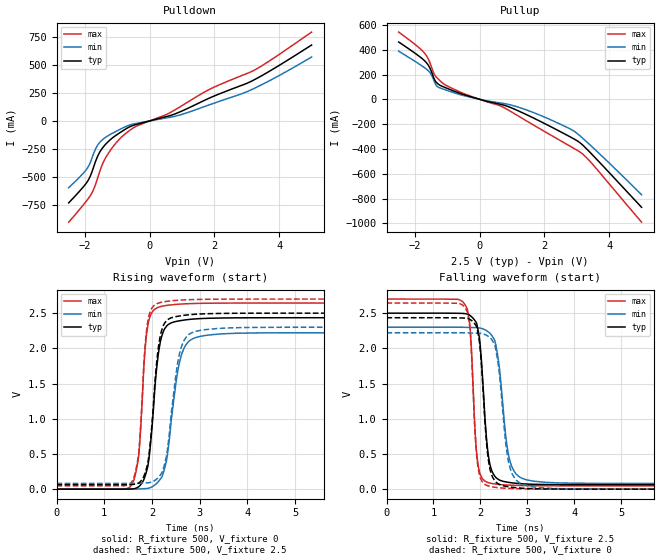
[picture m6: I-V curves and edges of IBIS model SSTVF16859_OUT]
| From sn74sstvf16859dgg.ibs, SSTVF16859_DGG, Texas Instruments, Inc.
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[Model]   SSTVF16859_OUT
Model_type  Output
Vref =   0
Rref =   500
Cref =   30p
Vmeas =   1.25
| variable   typ   min   max
C_comp   3.96pF   0.40pF   6.75pF
| C_pullup   3.64pF   0.40pF   6.75pF
| C_pulldown   4.29pF   2.35pF   5.77pF
[Temperature Range]   40   85   0
| Ambient temperature   25   70   0
[Voltage range]   2.5   2.3   2.7
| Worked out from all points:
|   slope of the pulldown table from 0 to 0.375 V, typ, clamps not added: 13.2 ohm
|   slope of the pullup table from 0 to 0.375 V, typ, clamps not added: 14.9 ohm
|   rising waveform, R_fixture 500, V_fixture 0: 20-80 % time 194ps typ, 256ps min, 144ps max; typ from 0 V to 2.44 V
|   falling waveform, R_fixture 500, V_fixture 2.5: 20-80 % time 156ps typ, 211ps min, 119ps max; typ from 2.5 V to 0.063 V
|   rising waveform, R_fixture 500, V_fixture 2.5: 20-80 % time 187ps typ, 239ps min, 142ps max; typ from 0.063 V to 2.5 V
|   falling waveform, R_fixture 500, V_fixture 0: 20-80 % time 155ps typ, 205ps min, 119ps max; typ from 2.44 V to 0 V
[Pulldown]
| SSTVF16859_OUT
|   Voltage   I(typ)   I(min)   I(max)
-2.5V     -732mA     -596.8mA   -904.7mA
-1.905V   -533.6mA   -413.3mA   -697.5mA
-1.725V   -407.4mA   -288.3mA   -608.5mA
-1.525V   -271.1mA   -186.6mA   -438mA
-1.215V   -167.6mA   -120.4mA   -263.3mA
-720mV    -68.68mA   -47.92mA   -107.3mA
-405mV    -31.09mA   -21.89mA   -46.25mA
935mV     80.65mA    53.1mA     125.3mA
1.84V     203.5mA    143.7mA    281mA
2.855V    319.5mA    243.8mA    406.9mA
3.48V     407.3mA    326.4mA    495.7mA
5V        678.2mA    571.1mA    793.7mA
[Pullup]
| SSTVF16859_OUT
|   Voltage   I(typ)   I(min)   I(max)
-2.5V     462.1mA    388.2mA    541.8mA
-1.72V    315.6mA    258.5mA    377.6mA
-1.52V    242.9mA    210.1mA    284.3mA
-1.355V   142.5mA    119.4mA    184.8mA
-1.095V   98.22mA    79.55mA    121.5mA
-455mV    34.94mA    27.86mA    42.59mA
715mV     -44.8mA    -32.33mA   -61.98mA
1.625V    -145.9mA   -103.1mA   -201.5mA
2.865V    -312.4mA   -248.6mA   -388.9mA
3.15V     -361.4mA   -306.3mA   -434.6mA
3.41V     -428.1mA   -367.8mA   -500.6mA
5V        -870.5mA   -768.8mA   -990.2mA
[Ramp]
| SSTVF16859_OUT
| variable   typ   min   max
dV/dt_r   1.46/2.01E-10   1.33/2.59E-10   1.59/1.46E-10
dV/dt_f   1.46/1.64E-10   1.33/2.22E-10   1.59/1.25E-10
R_load = 500
[Rising Waveform]
| SSTVF16859_OUT
R_fixture =   500
C_fixture =   0
L_fixture =   0
V_fixture =   0
V_fixture_min = 0
V_fixture_max = 0
|   Time   V(typ)   V(min)   V(max)
0s        6.564nV    7.235nV    33.42nV
1.575ns   3.4mV      334.3uV    66.37mV
1.72ns    33.25mV    2.581mV    462.2mV
1.845ns   164mV      6.949mV    1.888V
1.925ns   375.3mV    11.84mV    2.365V
2.125ns   1.877V     100.9mV    2.581V
2.29ns    2.3V       361.4mV    2.608V
2.625ns   2.397V     1.92V      2.63V
3.195ns   2.427V     2.19V      2.641V
24.99ns   2.435V     2.222V     2.644V
[Falling Waveform]
| SSTVF16859_OUT
R_fixture =   500
C_fixture =   0
L_fixture =   0
V_fixture =   2.5
V_fixture_min = 2.3
V_fixture_max = 2.7
|   Time   V(typ)   V(min)   V(max)
0s        2.5V       2.3V       2.7V
1.685ns   2.492V     2.299V     2.604V
1.78ns    2.466V     2.297V     2.286V
1.95ns    2.256V     2.291V     345.1mV
2.14ns    639.9mV    2.246V     99.72mV
2.255ns   239.8mV    2.169V     79.41mV
2.375ns   141.2mV    1.862V     68.76mV
2.64ns    92.86mV    374.5mV    56.6mV
3.145ns   69.07mV    112.8mV    49.13mV
24.99ns   62.81mV    81.57mV    47.07mV
[Rising Waveform]
| SSTVF16859_OUT
R_fixture =   500
C_fixture =   0
L_fixture =   0
V_fixture =   2.5
V_fixture_min = 2.3
V_fixture_max = 2.7
|   Time   V(typ)   V(min)   V(max)
0s        62.81mV    81.57mV    47.07mV
1.58ns    66.4mV     81.95mV    108.4mV
1.72ns    85.34mV    84.16mV    492.9mV
1.85ns    218.4mV    88.44mV    1.979V
1.925ns   422.2mV    91.33mV    2.426V
2.125ns   1.964V     160.6mV    2.641V
2.28ns    2.372V     396.3mV    2.664V
2.605ns   2.463V     1.996V     2.686V
3.11ns    2.491V     2.265V     2.696V
24.99ns   2.5V       2.3V       2.7V
[Falling Waveform]
| SSTVF16859_OUT
R_fixture =   500
C_fixture =   0
L_fixture =   0
V_fixture =   0
V_fixture_min = 0
V_fixture_max = 0
|   Time   V(typ)   V(min)   V(max)
0s        2.435V     2.222V     2.644V
1.69ns    2.428V     2.22V      2.555V
1.78ns    2.409V     2.219V     2.249V
1.95ns    2.207V     2.214V     303.4mV
2.14ns    581.6mV    2.182V     52.47mV
2.255ns   176.1mV    2.108V     32.18mV
2.375ns   77.81mV    1.788V     21.55mV
2.62ns    31.69mV    328.1mV    10.06mV
3.135ns   6.435mV    31.36mV    2.125mV
24.99ns   -51.95nV   -20.81nV   3.954nV
